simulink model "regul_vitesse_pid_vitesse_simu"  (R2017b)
settings: Solver=VariableStepAuto  StartTime=0.0  StopTime=10.0  RelTol=1e-3
libraries: simulink x1

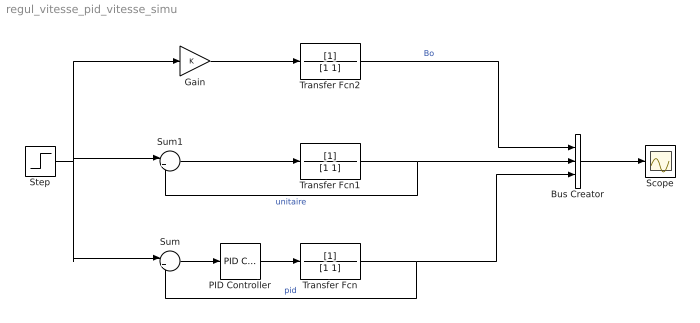
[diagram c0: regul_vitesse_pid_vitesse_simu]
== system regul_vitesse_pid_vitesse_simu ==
  Bus Creator : BusCreator  Inputs=3
  Gain : Gain
  PID Controller : simulink/Continuous/PID Controller  Controller=PID  Form=Parallel  TimeDomain=Continuous-time  SampleTime=-1  IntegratorMethod=Forward Euler  FilterMethod=Forward Euler  ControllerParametersSource=internal  P=0.912289474128758  I=1.34405253374515  D=0  UseFilter=on  N=100  TunerSelectOption=Transfer Function Based (PID Tuner App)  InitialConditionSource=internal  InitialConditionForIntegrator=0  InitialConditionForFilter=0  DifferentiatorICPrevScaledInput=0  ExternalReset=none  TrackingMode=off  Kt=1  LimitOutput=off  UpperSaturationLimit=inf  LowerSaturationLimit=-inf  LinearizeAsGain=on  AntiWindupMode=none  Kb=1  POutMin=[]  POutMax=[]  IOutMin=[]  IOutMax=[]  DOutMin=[]  DOutMax=[]  NOutMin=[]  NOutMax=[]  SumOutMin=[]  SumOutMax=[]  SaturationOutMin=[]  SaturationOutMax=[]  PParamMin=[]  PParamMax=[]  IParamMin=[]  IParamMax=[]  DParamMin=[]  DParamMax=[]  NParamMin=[]  NParamMax=[]  KbParamMin=[]  KbParamMax=[]  KtParamMin=[]  KtParamMax=[]  KbOutMin=[]  KbOutMax=[]  KtOutMin=[]  KtOutMax=[]  IntegratorOutMin=[]  IntegratorOutMax=[]  FilterOutMin=[]  FilterOutMax=[]  SumI1OutMin=[]  SumI1OutMax=[]  SumI2OutMin=[]  SumI2OutMax=[]  SumI3OutMin=[]  SumI3OutMax=[]  SumDOutMin=[]  SumDOutMax=[]  DifferentiatorOutMin=[]  DifferentiatorOutMax=[]  FilterDiffOutCoefMin=[]  FilterDiffOutCoefMax=[]  ReciprocalOutMin=[]  ReciprocalOutMax=[]  SumDenOutMin=[]  SumDenOutMax=[]  SumNumOutMin=[]  SumNumOutMax=[]  DivideOutMin=[]  DivideOutMax=[]  IntegratorContinuousStateAttributes=''  IntegratorStateMustResolveToSignalObject=off  IntegratorRTWStateStorageClass=Auto  FilterContinuousStateAttributes=''  FilterStateMustResolveToSignalObject=off  FilterRTWStateStorageClass=Auto
  Scope : Scope
  Step : Step  SampleTime=0
  Sum : Sum  Inputs=|+-
  Sum1 : Sum  Inputs=|+-
  Transfer Fcn : TransferFcn  Denominator=[1 1]
  Transfer Fcn1 : TransferFcn  Denominator=[1 1]
  Transfer Fcn2 : TransferFcn  Denominator=[1 1]
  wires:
  PID Controller/1 -> Transfer Fcn/1
  Sum/1 -> PID Controller/1
  Transfer Fcn/1 -> Bus Creator/3, Sum/2  "pid"
  Sum1/1 -> Transfer Fcn1/1
  Transfer Fcn1/1 -> Bus Creator/2, Sum1/2  "unitaire"
  Bus Creator/1 -> Scope/1
  Transfer Fcn2/1 -> Bus Creator/1  "Bo"
  Step/1 -> Sum1/1, Gain/1, Sum/1
  Gain/1 -> Transfer Fcn2/1
